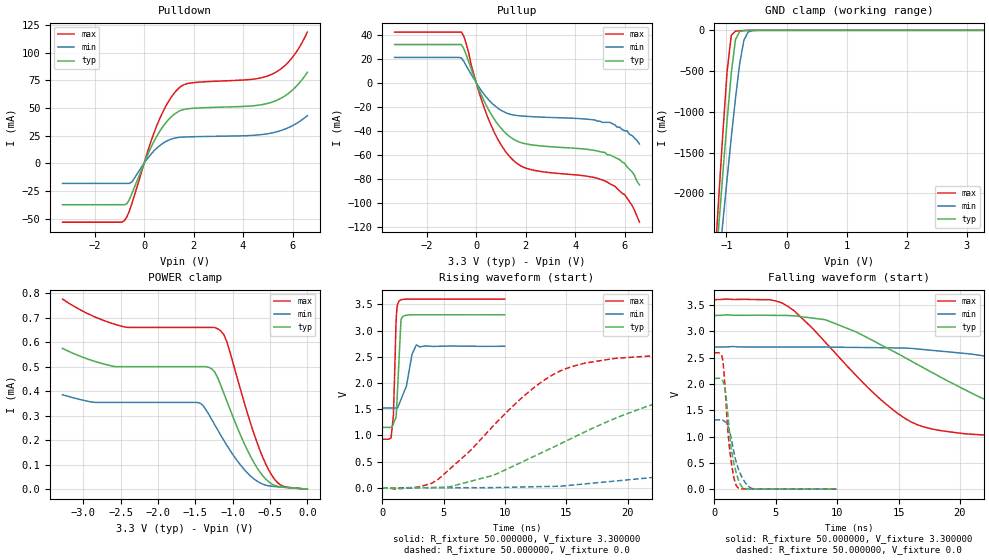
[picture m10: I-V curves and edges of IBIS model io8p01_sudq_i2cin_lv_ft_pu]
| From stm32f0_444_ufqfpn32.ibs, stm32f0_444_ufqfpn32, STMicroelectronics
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|   Model io8p01_sudq_i2cin_lv_ft_pu
[Model]  io8p01_sudq_i2cin_lv_ft_pu
Model_type I/O
Polarity   Non-Inverting
Enable   Active-Low
Vinl =   0.990000V
Vinh =   2.310000V
Vmeas =  1.650000V
Cref =   50.000000pF
Rref =   100.000000M
Vref =   0.0V
C_comp   2.070000pF   1.996000pF   2.160200pF
[Temperature Range]   25.000000   0.125000k   -40.000000
[Pullup Reference]   3.300000V   2.700000V   3.600000V
[Pulldown Reference]   0.0V   0.0V   0.0V
[POWER Clamp Reference]   3.300000V   2.700000V   3.600000V
[GND Clamp Reference]   0.0V   0.0V   0.0V
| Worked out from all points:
|   slope of the pulldown table from 0 to 0.495 V, typ, clamps not added: 20.9 ohm
|   slope of the pullup table from 0 to 0.495 V, typ, clamps not added: 22.2 ohm
|   GND clamp passes 1 mA (typ) near -0.64 V on its own axis
|   rising waveform, R_fixture 50.000000, V_fixture 3.300000: 20-80 % time 271ps typ, 710ps min, 190ps max; typ from 1.15 V to 3.3 V
|   rising waveform, R_fixture 50.000000, V_fixture 0.0: 20-80 % time 12.6ns typ, 30.7ns min, 7.05ns max; typ from 0.001 V to 2.1 V
|   falling waveform, R_fixture 50.000000, V_fixture 3.300000: 20-80 % time 10.9ns typ, 22.9ns min, 6.87ns max; typ from 3.3 V to 1.15 V
|   falling waveform, R_fixture 50.000000, V_fixture 0.0: 20-80 % time 670ps typ, 882ps min, 550ps max; typ from 2.1 V to 0.001 V
[Pulldown]
|Voltage   I(typ)   I(min)   I(max)
-3.3V     -37.45mA   -18.2mA    -53.24mA
-800mV    -37.45mA   -18.2mA    -51.9mA
-700mV    -36.7mA    -18.2mA    -48.48mA
-500mV    -27.71mA   -17.01mA   -36.66mA
500mV     23.91mA    13.38mA    33.24mA
900mV     37.17mA    19.88mA    52.48mA
1.3V      45.55mA    23.01mA    65.5mA
1.8V      49.29mA    23.83mA    72.18mA
4.4V      51.88mA    25.21mA    75.91mA
5.2V      55.41mA    27.53mA    80.72mA
5.9V      64.2mA     32.82mA    93.01mA
6.6V      82.13mA    42.97mA    118.5mA
[Pullup]
|Voltage   I(typ)   I(min)   I(max)
-3.3V     31.7mA     20.96mA    42.04mA
-600mV    31.7mA     20.58mA    42.04mA
-400mV    22.99mA    13.87mA    32.11mA
0V        90fA       16pA       0A
500mV     -22.5mA    -14.16mA   -30.52mA
900mV     -35.28mA   -21.54mA   -48mA
1.4V      -45.54mA   -26.4mA    -62.54mA
2.2V      -51.57mA   -28.22mA   -72.25mA
5.3V      -60mA      -33mA      -82.7mA
6V        -67mA      -40mA      -93mA
6.3V      -74mA      -44mA      -102mA
6.6V      -85mA      -51mA      -116mA
[GND_clamp]
|Voltage   I(typ)   I(min)   I(max)
-3.3V     -9.366A    -9.678A    -9.859A
-1.2V     -3.091A    -3.431A    -2.911A
-1.13V    -2.415A    -2.888A    -2.072A
-1.06V    -1.751A    -2.352A    -1.259A
-990mV    -1.112A    -1.826A    -509.3mA
-920mV    -522.9mA   -1.315A    -61.61mA
-850mV    -112.5mA   -833.8mA   -10.22mA
-780mV    -13.59mA   -408.1mA   -5.256mA
-710mV    -3.081mA   -122.1mA   -2.635mA
-640mV    -945.2uA   -21.36mA   -905.7uA
-570mV    -199.6uA   -4.142mA   -156.8uA
3.28V     0A         0A         0A
[POWER_clamp]
|Voltage   I(typ)   I(min)   I(max)
-3.28V    574uA      385.1uA    775.2uA
-2.88V    524.3uA    354.9uA    706.9uA
-2.44V    499.5uA    353.8uA    660.7uA
-1.44V    499.5uA    351.5uA    659.5uA
-1.28V    490.2uA    283.5uA    659.5uA
-1.16V    423.6uA    220uA      645uA
-1.08V    360.3uA    179.6uA    602.6uA
-800mV    157uA      65.19uA    307.1uA
-640mV    71.83uA    26.55uA    162.4uA
-520mV    30.52uA    13.8uA     79.51uA
-360mV    9.625uA    8.656uA    17.31uA
0V        0A         0A         0A
[Ramp]
| variable   typ   min   max
dV/dt_r  1.26192/12.62993n   0.78964/30.68305n   1.55415/7.03902n
dV/dt_f  1.28874/10.84459n   0.70548/22.82726n   1.60395/6.85369n
R_load = 50.000000
[Rising Waveform]
R_fixture= 50.000000
V_fixture= 3.300000
V_fixture_min= 2.700000
V_fixture_max= 3.600000
|time   V(typ)   V(min)   V(max)
0s        1.152V     1.524V     926.8mV
720.7ps   1.154V     1.523V     979.6mV
900.9ps   1.223V     1.522V     1.384V
1.121ns   1.348V     1.523V     3.185V
1.201ns   1.704V     1.523V     3.444V
1.361ns   2.463V     1.596V     3.562V
1.522ns   3.206V     1.688V     3.586V
2.422ns   3.3V       2.548V     3.599V
2.783ns   3.3V       2.726V     3.599V
9.97ns    3.3V       2.7V       3.6V
[Rising Waveform]
R_fixture= 50.000000
V_fixture= 0.0
V_fixture_min= 0.0
V_fixture_max= 0.0
|time   V(typ)   V(min)   V(max)
0s        1.1mV      1.225mV    1.052mV
4.505ns   9.679mV    3.246mV    153.6mV
9.009ns   237.3mV    4.967mV    1.175V
12.01ns   563.9mV    19.45mV    1.847V
14.51ns   841.5mV    31.75mV    2.232V
24.02ns   1.725V     241.7mV    2.547V
38.04ns   2.052V     644.7mV    2.589V
52.05ns   2.095V     993.9mV    2.592V
69.07ns   2.104V     1.204V     2.592V
249.2ns   2.104V     1.317V     2.592V
[Falling Waveform]
R_fixture= 50.000000
V_fixture= 3.300000
V_fixture_min= 2.700000
V_fixture_max= 3.600000
|time   V(typ)   V(min)   V(max)
0s        3.3V       2.7V       3.6V
6.006ns   3.299V     2.701V     3.47V
9.009ns   3.22V      2.7V       2.798V
13.01ns   2.81V      2.689V     1.817V
16.02ns   2.436V     2.675V     1.279V
24.52ns   1.502V     2.444V     991.9mV
31.03ns   1.3V       2.21V      957.5mV
45.55ns   1.193V     1.774V     932mV
74.57ns   1.155V     1.574V     926.9mV
249.2ns   1.152V     1.524V     926.8mV
[Falling Waveform]
R_fixture= 50.000000
V_fixture= 0.0
V_fixture_min= 0.0
V_fixture_max= 0.0
|time   V(typ)   V(min)   V(max)
0s        2.104V     1.317V     2.592V
660.7ps   2.063V     1.316V     2.468V
900.9ps   1.844V     1.274V     1.809V
1.081ns   1.441V     1.207V     1.142V
1.221ns   1.088V     1.115V     792.3mV
1.562ns   519.1mV    733.7mV    249.9mV
1.862ns   243.5mV    450.6mV    41.25mV
2.342ns   26.13mV    186.6mV    7.039mV
3.123ns   3.191mV    11.11mV    4.635mV
9.97ns    1.1mV      1.225mV    1.052mV
